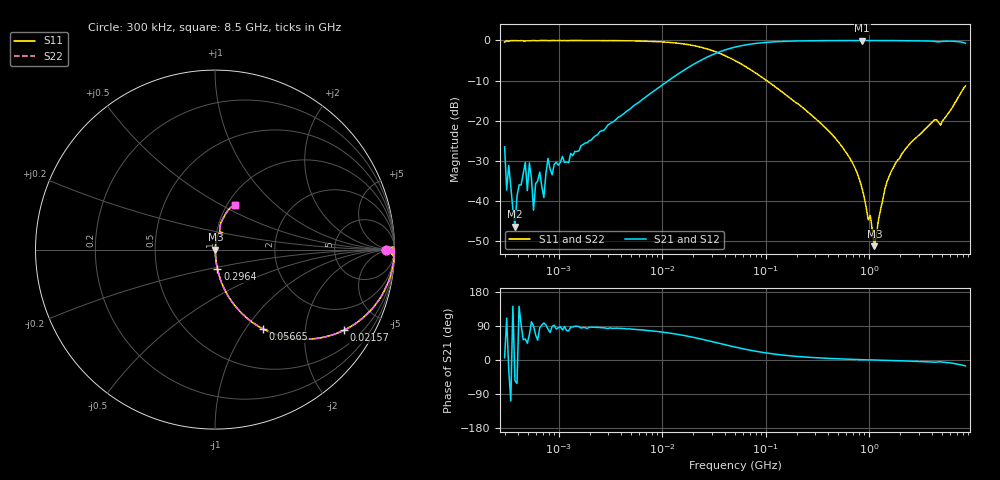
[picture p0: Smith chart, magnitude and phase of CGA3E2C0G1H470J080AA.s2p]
! S-parameter Generated by TDK Corporation
! Copyright(C) 2015 TDK Corporation.
! All Rights Reserved.
! TDK P/N: CGA3E2C0G1H470J080AA (Multilayer Ceramic Chip Capacitors)
! Property: C=47pF
! Size(LxWxT): 1.6x0.8x0.8mm, 0.063x0.031x0.031inches
! Model Type: s2p (Touchstone File Format Version 1.0)
! Frequency: DC=Yes Start=0.3MHz Stop=8500MHz 225points Log-sweep
! Note:
! Model Generated on Jun. 23, 2015
! Hash(MD5):
! Port Assignments:
!  1 ---| |--- 2
! Applicable Conditions:
!  Temperature = 25 degC
!  DC Bias Voltage = 0 V
!  Small Signal Operation
! Terms and conditions regarding TDK Simulation Models
! (1)This simulation model is being provided solely for informational purposes. Please refer to the specifications of the products in terms of detailed characteristics of such products.
! (2)In no event shall TDK Corporation of any of its subsidiaries be liable for any loss or damage arising, directly or indirectly,
!  From any information contained in this simulation model, including, but not limited to loss or damages arising from any inaccuracies, omissions or errors in connection with such information.
! (3)Any and all copyrights on this simulation model are owned by TDK Corporation.
!  Duplication or redistribution of this simulation model without prior written permission from TDK Corporation is prohibited.
! (4)This simulation model is subject to any modification or change without any prior notice.
! (5)Neither TDK Corporation nor any of its subsidiaries shall make any warranty, express or implied,
!  Including but not limited to the correctness, implied warranties of merchantability and fitness for a particular purpose with respect to this simulation models.
! (6)The use of this simulation model shall be deemed to have consented to the terms and conditions hereof.
# MHz S MA R 50
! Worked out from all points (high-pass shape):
!   224 points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, 300 kHz to 8.5 GHz, reference 50 ohm
!   highest |S21| = -0.02 dB at 853.4 MHz (marker M1); lowest = -46.4 dB at 377.5 kHz (marker M2)
!   |S21| within 3 dB of the highest: 34.34 MHz to end of sweep
!   lowest |S11| = -51.3 dB at 1.124 GHz (marker M3), VSWR 1.01, Z = 50.3 - j0.0822 ohm
!   |S11| at or under -10 dB: 102.1 MHz to end of sweep
!   |S22| runs from -51.3 to 0.0 dB; largest |S21 - S12| = 5.9e-12
!   S11 on the Smith chart (normalised r, x): 300 kHz: 41, -4; 21.57 MHz: 1.00, -3.19; 56.65 MHz: 1.00, -1.21; 296.4 MHz: 1.00, -0.22; 8.5 GHz: 1.08, +0.58
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0.3  0.9529 -0.3  0.04738 6.0  0.04738 6.0  0.9529 -0.3
0.3141136  0.995 -0.7  0.01367 110.4  0.01367 110.4  0.995 -0.7
0.3288911  0.9752 0.7  0.02769 -26.2  0.02769 -26.2  0.9752 0.7
0.3775275  0.9972 0.1  0.004772 -54.2  0.004772 -54.2  0.9972 0.1
0.47509  0.9832 -1.4  0.03021 55.4  0.03021 55.4  0.9832 -1.4
0.4974407  0.9904 -0.5  0.01344 44.3  0.01344 44.3  0.9904 -0.5
0.5208429  0.989 -1.6  0.02983 67.5  0.02983 67.5  0.989 -1.6
0.5710021  1 -0.4  0.007669 89.7  0.007669 89.7  1 -0.4
0.6554417  0.9982 -1.3  0.02288 84.9  0.02288 84.9  0.9982 -1.3
0.7185633  0.9983 -0.6  0.011 97.8  0.011 97.8  0.9983 -0.6
0.7877636  0.9954 -1.9  0.03385 81.5  0.03385 81.5  0.9954 -1.9
1.72111  0.9975 -2.9  0.0505 85.7  0.0505 85.7  0.9975 -2.9
9.430415  0.9638 -15.3  0.2642 74.5  0.2642 74.5  0.9638 -15.3
21.57293  0.8466 -32.1  0.5313 57.8  0.5313 57.8  0.8466 -32.1
51.67171  0.5528 -56.3  0.8324 33.6  0.8324 33.6  0.5528 -56.3
56.64789  0.5176 -58.7  0.8547 31.2  0.8547 31.2  0.5176 -58.7
283.1228  0.1147 -82.5  0.9915 6.6  0.9915 6.6  0.1147 -82.5
296.4424  0.1088 -82.8  0.9922 6.2  0.9922 6.2  0.1088 -82.8
853.3868  0.01436 -81.1  0.9979 0.8  0.9979 0.8  0.01436 -81.1
1124.446  0.002732 -17.4  0.9974 0.0  0.9974 0.0  0.002732 -17.4
1551.304  0.0198 80.5  0.9969 -1.1  0.9969 -1.1  0.0198 80.5
8500  0.2706 66.2  0.9247 -15.5  0.9247 -15.5  0.2706 66.2
